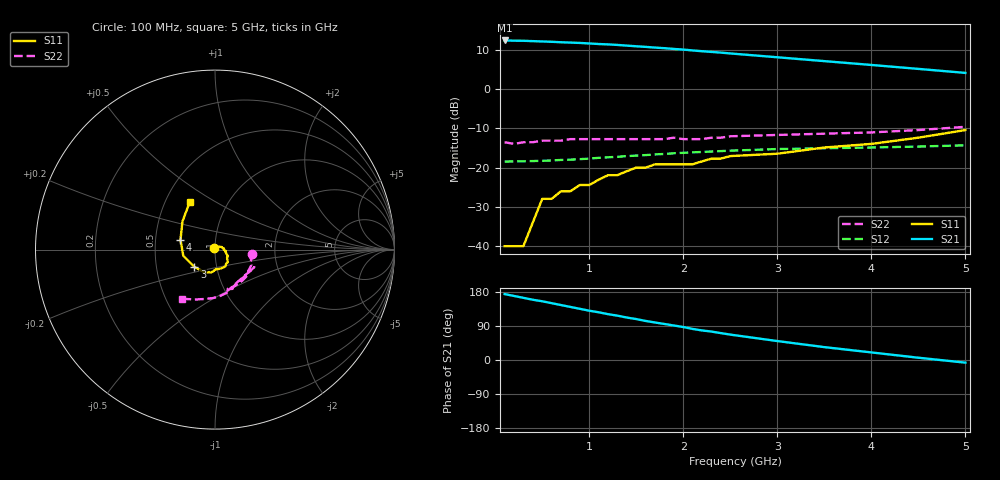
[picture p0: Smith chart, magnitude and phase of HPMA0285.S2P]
! HPMA-0285
! Typical S-Parameters, Z  = 50 , TA = 25 C, Id = 25mA
# ghz s ma r 50
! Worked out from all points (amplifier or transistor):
!   30 points, 100 MHz to 5 GHz, reference 50 ohm
!   highest |S21| = 12.3 dB at 100 MHz (marker M1)
!   |S21| within 3 dB of that: start of sweep to 2.348 GHz
!   unconditionally stable (mu >= 1): start of sweep to end of sweep
!   at 600 MHz: K = 1.22, MAG = 12.2 dB, |S12| = -18.2 dB
!   at 1.6 GHz: K = 1.21, MAG = 11.0 dB, |S12| = -16.8 dB
!   at 5 GHz: K = 1.37, MAG = 5.6 dB, |S12| = -14.3 dB
!   S11 on the Smith chart (normalised r, x): 100 MHz: 0.98, +0.01; 3 GHz: 0.78, -0.15; 4 GHz: 0.67, +0.08; 5 GHz: 0.66, +0.39
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0.1  0.01 141.0  4.14 174.0  0.119 1.0  0.21 -6.0
0.3  0.01 94.0  4.1 164.0  0.12 4.0  0.21 -16.0
0.4  0.02 64.0  4.06 159.0  0.121 5.0  0.21 -21.0
0.5  0.04 21.0  4.02 155.0  0.122 6.0  0.22 -23.0
0.8  0.05 -1.0  3.89 140.0  0.126 8.0  0.23 -36.0
0.9  0.06 -7.0  3.85 135.0  0.128 9.0  0.23 -41.0
1  0.06 -13.0  3.79 130.0  0.13 10.0  0.23 -45.0
1.2  0.08 -27.0  3.69 121.0  0.135 11.0  0.23 -51.0
1.4  0.09 -40.0  3.56 112.0  0.14 11.0  0.23 -57.0
1.6  0.1 -52.0  3.43 103.0  0.144 11.0  0.23 -61.0
1.8  0.11 -64.0  3.3 95.0  0.149 11.0  0.23 -65.0
2  0.11 -79.0  3.17 87.0  0.154 11.0  0.23 -68.0
2.1  0.11 -88.0  3.09 82.0  0.156 11.0  0.23 -71.0
2.2  0.12 -94.0  3.02 78.0  0.158 10.0  0.23 -72.0
2.3  0.13 -100.0  2.96 75.0  0.16 10.0  0.24 -73.0
2.4  0.13 -105.0  2.9 71.0  0.162 10.0  0.24 -24.0
2.5  0.14 -112.0  2.83 67.0  0.164 9.0  0.25 -75.0
3  0.15 -140.0  2.53 50.0  0.172 7.0  0.26 -84.0
3.5  0.18 -169.0  2.26 34.0  0.176 5.0  0.27 -92.0
4  0.2 164.0  2.02 20.0  0.18 4.0  0.28 -101.0
4.5  0.24 139.0  1.8 6.0  0.185 4.0  0.3 -112.0
5  0.3 118.0  1.6 -7.0  0.192 4.0  0.33 -124.0
